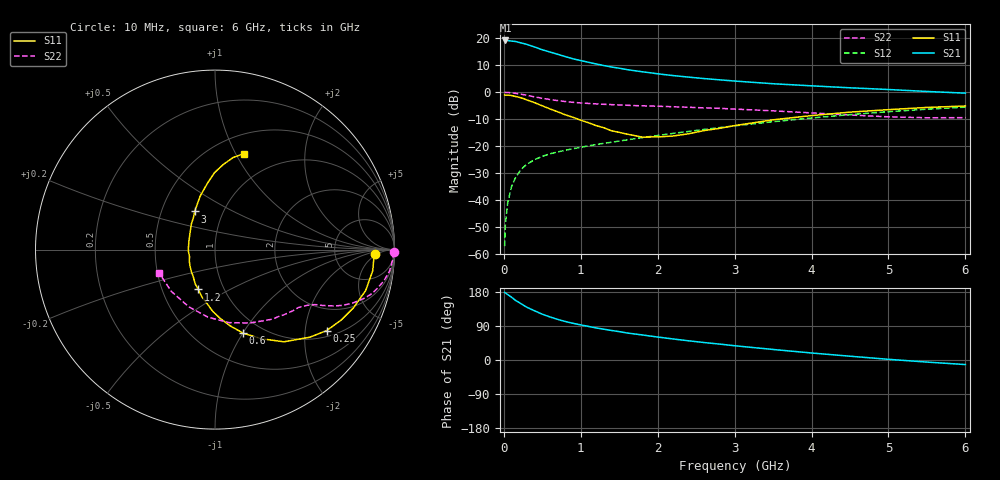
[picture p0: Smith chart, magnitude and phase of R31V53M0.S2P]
! SIEMENS Small Signal Semiconductors
! BFR181
! Si NPN RF Bipolar Junction Transistor in SOT23
! VCE = 1.5 V  IC = 3 mA
! Common Emitter S-Parameters:  May  1996
# GHz  S  MA  R  50
!  f  S11  S21  S12  S22
! GHz  MAG  ANG  MAG  ANG  MAG  ANG  MAG  ANG
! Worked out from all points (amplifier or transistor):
!   36 points, 10 MHz to 6 GHz, reference 50 ohm
!   highest |S21| = 19.2 dB at 20 MHz (marker M1)
!   |S21| within 3 dB of that: start of sweep to 456.3 MHz
!   unconditionally stable (mu >= 1): 1.318 GHz to 3.217 GHz
!   at 250 MHz: K = 0.31, MSG = 23.0 dB, |S12| = -27.9 dB
!   at 1.4 GHz: K = 1.02, MAG = 13.0 dB, |S12| = -18.5 dB
!   at 6 GHz: K = 0.87, MSG = 2.6 dB, |S12| = -5.5 dB
!   S11 on the Smith chart (normalised r, x): 10 MHz: 16, -4; 250 MHz: 1.18, -2.60; 600 MHz: 0.82, -1.01; 1.2 GHz: 0.76, -0.36; 3 GHz: 0.73, +0.33; 6 GHz: 0.70, +1.08
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0.01  0.8913 -1.6  9.04 178.7  0.0014 85.5  0.9951 -0.8
0.02  0.8863 -3.1  9.137 176.9  0.0036 88.2  0.9938 -1.5
0.05  0.8867 -7.6  9.107 172.7  0.0089 86.7  0.9904 -3.6
0.1  0.8699 -15.2  8.895 165.7  0.0178 82.1  0.98 -7.0
0.15  0.8365 -22.9  8.756 157.6  0.0258 77.0  0.9575 -10.4
0.25  0.7682 -36.0  8.049 145.2  0.0403 70.3  0.9074 -15.7
0.3  0.7195 -42.7  7.714 139.1  0.0464 67.9  0.8777 -17.9
0.4  0.6415 -53.2  6.924 129.8  0.0564 63.2  0.8217 -21.3
0.5  0.5607 -62.4  6.136 120.8  0.0649 61.2  0.7736 -23.7
0.6  0.4917 -71.3  5.571 113.6  0.0723 59.1  0.7345 -25.3
0.7  0.4342 -78.6  5.063 107.2  0.0782 57.7  0.7006 -26.5
0.8  0.3817 -86.1  4.581 101.5  0.0841 57.0  0.6733 -27.5
0.9  0.3434 -92.2  4.177 96.8  0.0898 56.9  0.6506 -28.2
1.1  0.2726 -105.6  3.597 88.6  0.1016 57.3  0.621 -29.7
1.2  0.2408 -112.9  3.35 84.6  0.1072 57.3  0.6087 -30.5
1.6  0.1676 -146.0  2.634 71.4  0.131 58.2  0.5741 -33.8
2.2  0.1546 159.2  2.038 55.5  0.1727 58.6  0.5384 -40.9
3  0.2409 118.0  1.616 37.6  0.2384 55.8  0.4883 -53.6
3.5  0.3085 105.6  1.439 27.8  0.2844 52.4  0.4524 -64.7
4.5  0.4283 90.4  1.21 10.0  0.3851 42.8  0.3786 -95.9
5.5  0.5234 78.8  1.035 -5.5  0.4851 30.0  0.3367 -136.2
6  0.5572 73.4  0.963 -12.0  0.5303 22.8  0.3381 -157.7
